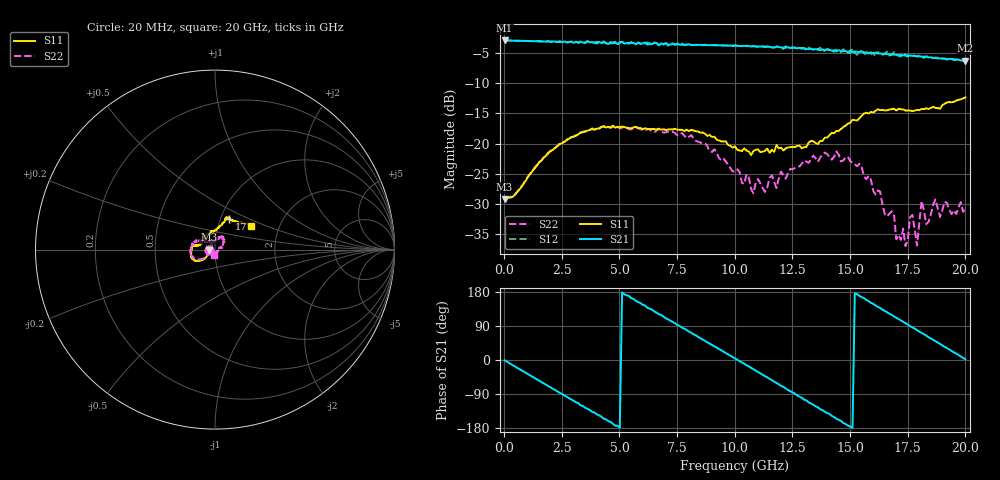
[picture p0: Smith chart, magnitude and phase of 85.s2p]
!Agilent Technologies,N5230A,US43500223,A.07.50.48
!Agilent N5230A: A.07.50.48
!Date: Thursday, September 17, 2015 18:58:51
!Correction: S11(Full 2 Port(1,2))
!S21(Full 2 Port(1,2))
!S12(Full 2 Port(1,2))
!S22(Full 2 Port(1,2))
!S2P File: Measurements: S11, S21, S12, S22:
# Hz S  dB  R 50
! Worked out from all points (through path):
!   201 points, 20 MHz to 20 GHz, reference 50 ohm
!   highest |S21| = -2.93 dB at 20 MHz (marker M1); lowest = -6.3 dB at 20 GHz (marker M2)
!   group delay of S21, straight-line fit = 99.5 ps
!   lowest |S11| = -29.2 dB at 20 MHz (marker M3), VSWR 1.07, Z = 46.7 - j0.0251 ohm
!   |S11| at or under -10 dB: start of sweep to end of sweep
!   |S22| runs from -37.0 to -17.2 dB; largest |S21 - S12| = 0.061
!   S11 on the Smith chart (normalised r, x): 20 MHz: 0.93, -0.00; 17 GHz: 1.10, +0.39; 20 GHz: 1.44, +0.40
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2e7  -29.24 -179.6  -2.93 -0.8  -2.93 -0.8  -29.03 179.4
1.9181e9  -21.55 -139.8  -3.06 -69.0  -3.06 -69.0  -21.55 -142.3
3.4166e9  -18.13 -150.1  -3.25 -121.5  -3.44 -121.8  -18.01 -155.8
5.1149e9  -17.18 -166.4  -3.12 178.6  -3.19 179.1  -17.37 -177.9
6.7133e9  -17.54 179.1  -3.76 120.7  -3.66 120.7  -17.55 165.2
8.012e9  -17.93 171.5  -3.54 75.0  -3.51 75.8  -18.89 155.1
1.001e10  -20.45 163.8  -3.79 4.1  -3.74 5.0  -24.61 130.3
1.08092e10  -21.22 156.1  -3.83 -24.5  -3.87 -23.3  -28.21 120.4
1.19081e10  -20.77 135.8  -4.03 -64.1  -3.93 -64.5  -25.83 87.9
1.34066e10  -19.63 97.9  -4.43 -118.3  -4.42 -119.7  -21.98 64.4
1.51049e10  -16.07 73.7  -4.88 -179.4  -4.26 179.8  -23.14 49.5
1.67033e10  -14.37 69.0  -5.23 122.0  -5.43 123.0  -31.62 -7.4
1.69031e10  -14.22 66.7  -5.28 115.1  -4.89 119.9  -31.69 -2.2
1.7003e10  -14.52 65.3  -5.31 111.5  -5.21 110.6  -35.84 -35.1
1.74026e10  -14.53 64.9  -5.45 97.2  -5.36 97.3  -36.98 -46.9
1.77023e10  -14.62 59.9  -5.48 85.8  -5.36 87.2  -31.82 -78.4
1.79021e10  -14.42 58.2  -5.53 78.7  -5.62 81.7  -36.88 -86.3
1.81019e10  -14.28 55.3  -5.62 71.6  -5.51 72.7  -29.49 -101.2
1.83017e10  -14.17 54.5  -5.64 64.4  -5.54 66.7  -33.32 -91.6
1.87013e10  -14.08 47.4  -5.78 49.6  -5.80 51.7  -29.25 -95.1
1.89011e10  -14.26 48.3  -5.92 42.3  -5.97 44.3  -32.16 -124.4
2e10  -12.36 33.0  -6.29 2.3  -6.27 4.5  -30.75 -97.8
